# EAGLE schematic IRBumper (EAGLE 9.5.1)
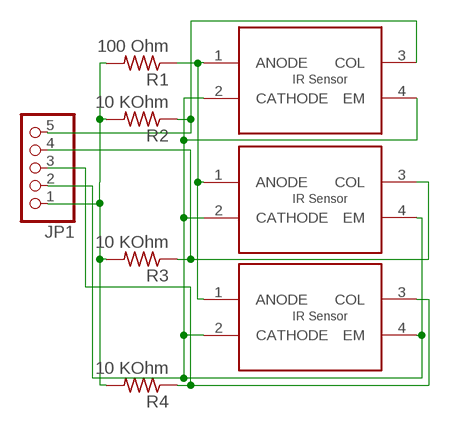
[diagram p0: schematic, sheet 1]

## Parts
JP1  PINHD-1X5  [1X05]
R1  100 Ohm  R-US_M0805  [M0805]
R2  10 KOhm  R-US_M0805  [M0805]
R3  10 KOhm  R-US_M0805  [M0805]
R4  10 KOhm  R-US_M0805  [M0805]
U$1  QRE1113GR  [4-SMD]
U$2  QRE1113GR  [4-SMD]
U$3  QRE1113GR  [4-SMD]

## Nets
GND: JP1.2 U$1.2(CATHODE) U$1.4(EM) U$2.2(CATHODE) U$2.4(EM) U$3.2(CATHODE) U$3.4(EM)
N$1: R1.1 U$1.1(ANODE) U$2.1(ANODE) U$3.1(ANODE)
N$2: JP1.5 R2.1 U$2.3(COL)
N$5: JP1.4 R3.1 U$1.3(COL)
N$6: JP1.3 R4.1 U$3.3(COL)
VDD_5: JP1.1 R1.2 R2.2 R3.2 R4.2

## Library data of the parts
JP1 = pinhead:PINHD-1X5: PIN HEADER
R1-R4 = rcl:R-US_: RESISTOR, American symbol; SPICEPREFIX: R
U$1-U$3 = MILESTONE4LIB_E:QRE1113GR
